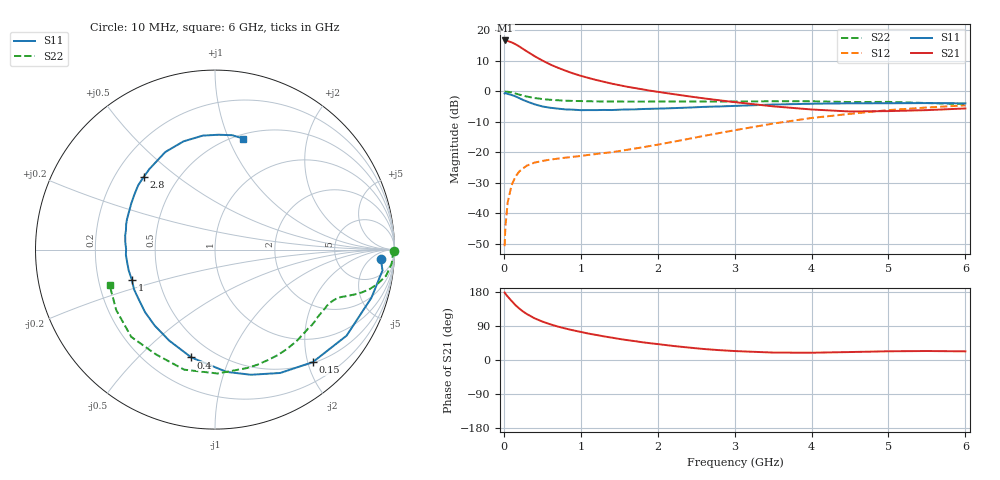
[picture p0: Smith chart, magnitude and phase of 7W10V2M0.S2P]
! Infineon Technologies  Discrete & RF Semiconductors
! BFS17W
! Si NPN RF Bipolar Junction Transistor in SOT323
! VCE = 10 V  IC = 2 mA
! Common Emitter S-Parameters:  August  1999
# GHz  S  MA  R  50
!  f  S11  S21  S12  S22
! GHz  MAG  ANG  MAG  ANG  MAG  ANG  MAG  ANG
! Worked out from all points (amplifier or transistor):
!   36 points, 10 MHz to 6 GHz, reference 50 ohm
!   highest |S21| = 16.7 dB at 20 MHz (marker M1)
!   |S21| within 3 dB of that: start of sweep to 263.4 MHz
!   unconditionally stable (mu >= 1): 864.8 MHz to 2.629 GHz; 4.488 GHz to end of sweep
!   at 250 MHz: K = 0.35, MSG = 19.6 dB, |S12| = -25.2 dB
!   at 1.4 GHz: K = 1.25, MAG = 8.2 dB, |S12| = -19.9 dB
!   at 6 GHz: K = 1.07, MAG = -2.1 dB, |S12| = -4.6 dB
!   S11 on the Smith chart (normalised r, x): 10 MHz: 17, -12; 150 MHz: 0.52, -2.09; 400 MHz: 0.38, -0.73; 1 GHz: 0.35, -0.16; 2.8 GHz: 0.32, +0.38; 6 GHz: 0.54, +1.13
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0.01  0.9257 -3.3  6.826 178.0  0.0029 90.3  0.9994 -0.4
0.02  0.9404 -7.1  6.858 174.9  0.006 89.3  0.9909 -1.8
0.05  0.9119 -17.1  6.719 167.4  0.0151 81.3  0.9875 -4.6
0.1  0.876 -33.2  6.388 156.0  0.0288 72.5  0.9641 -8.7
0.15  0.8306 -49.0  5.966 145.0  0.0398 64.3  0.9244 -12.0
0.2  0.7777 -62.1  5.475 135.9  0.0486 59.3  0.8882 -14.4
0.25  0.7254 -74.0  4.978 128.0  0.0548 54.0  0.8533 -16.2
0.3  0.6844 -84.6  4.534 121.2  0.0608 50.9  0.8246 -17.5
0.4  0.615 -102.4  3.786 110.0  0.0681 46.2  0.7795 -19.4
0.5  0.5678 -116.6  3.221 101.5  0.0724 43.8  0.7508 -20.6
0.6  0.5406 -128.4  2.779 94.4  0.0762 43.3  0.7304 -21.9
0.7  0.5229 -138.2  2.454 88.4  0.079 43.7  0.7171 -23.3
0.8  0.5075 -146.7  2.194 83.1  0.082 44.3  0.7063 -24.8
1  0.4932 -159.7  1.804 74.1  0.0875 47.2  0.6952 -27.9
1.1  0.4946 -166.3  1.665 69.7  0.0911 49.0  0.6904 -29.9
1.6  0.5067 170.9  1.196 52.6  0.1102 58.5  0.6802 -40.2
2.2  0.5322 151.4  0.906 37.1  0.1493 68.0  0.6834 -54.3
2.8  0.5673 134.5  0.716 26.0  0.2076 71.6  0.6835 -69.8
3.5  0.6102 117.0  0.57 19.6  0.2971 69.4  0.6904 -88.8
4.5  0.6387 96.1  0.469 21.0  0.4287 57.8  0.6701 -119.5
5.5  0.6444 81.4  0.494 23.7  0.5454 44.0  0.6453 -148.5
6  0.6382 75.7  0.526 22.8  0.5904 37.2  0.6194 -161.6
